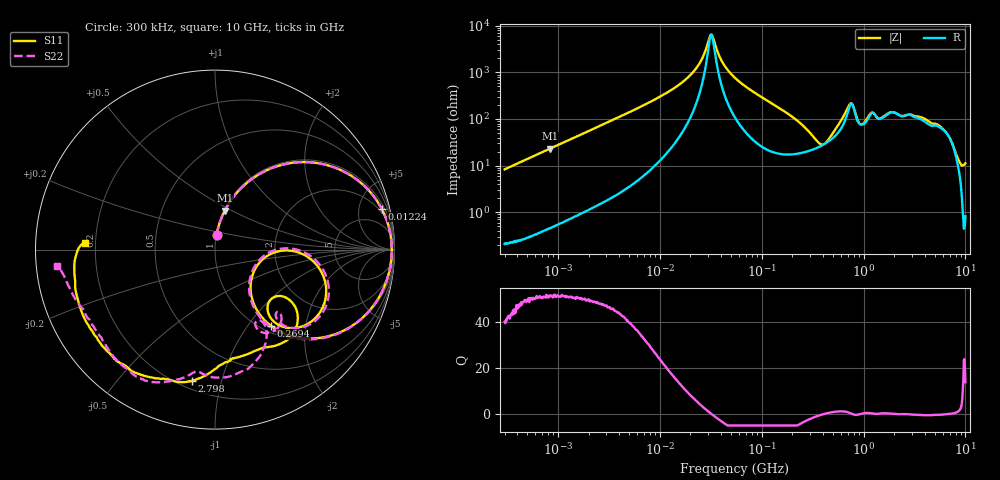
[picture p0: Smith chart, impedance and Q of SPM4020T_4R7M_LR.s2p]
! S-Parameter Data Generated by TDK Corporation
! Copyright(C) 2019 TDK Corporation.
! All Rights Reserved.
! TDK P/N: SPM4020T-4R7M-LR (Inductor)
! Property: L=4.7uH at 100kHz
! Size(LxWxT): 4.4x4.1x2mm
! Model Type: s2p (Touchstone File Format Version 1.0)
! Frequency: DC=Yes Start=0.3MHz Stop=10000MHz 802points Log-sweep
! Model Generated on Sep. 23, 2019
! Port Assignments:
!  1 ---@@@--- 2
! Applicable Conditions:
!  Temperature = 25 degC
!  DC Bias Current = 0 A
!  Small Signal Operation
! Terms and conditions regarding TDK Simulation Models
! (1)This simulation model is being provided solely for informational purposes. Please refer to the specifications of the products in terms of detailed characteristics of such products.
! (2)In no event shall TDK Corporation of any of its subsidiaries be liable for any loss or damage arising, directly or indirectly,
!  From any information contained in this simulation model, including, but not limited to loss or damages arising from any inaccuracies, omissions or errors in connection with such information.
! (3)Any and all copyrights on this simulation model are owned by TDK Corporation.
!  Duplication or redistribution of this simulation model without prior written permission from TDK Corporation is prohibited.
! (4)This simulation model is subject to any modification or change without any prior notice.
! (5)Neither TDK Corporation nor any of its subsidiaries shall make any warranty, express or implied,
!  Including but not limited to the correctness, implied warranties of merchantability and fitness for a particular purpose with respect to this simulation models.
! (6)The use of this simulation model shall be deemed to have consented to the terms and conditions hereof.
# Hz S MA R 50
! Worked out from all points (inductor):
!   801 points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, 300 kHz to 10 GHz, reference 50 ohm
!   read as one part in series: L = 4.4 uH near 318.3 kHz
!   highest Q = 51.2 at 832.9 kHz (marker M1), where L = 4.4 uH
!   self-resonance near 32.06 MHz
!   S11 on the Smith chart (normalised r, x): 300 kHz: 1.00, +0.17; 12.24 MHz: 1.50, +7.98; 269.4 MHz: 1.10, -1.30; 2.798 GHz: 0.25, -0.81; 10 GHz: 0.16, +0.02
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300000  0.08244 83.8  0.9945 -4.8  0.9946 -4.8  0.08211 83.8
832928  0.2231 76.0  0.9704 -12.9  0.9705 -12.9  0.223 75.9
1713600  0.4229 63.8  0.8977 -25.1  0.8978 -25.1  0.4229 63.8
3911703  0.7253 42.1  0.6721 -46.6  0.6722 -46.6  0.7251 42.1
9671944  0.9328 18.5  0.3243 -69.1  0.3243 -69.1  0.9328 18.5
1.224117e7  0.956 13.8  0.2469 -73.1  0.2469 -73.2  0.956 13.8
2.220835e7  0.9824 4.1  0.08621 -76.6  0.08624 -76.7  0.9824 4.0
3.206042e7  0.9848 -1.2  0.01508 -2.2  0.01508 -2.2  0.9848 -1.2
5.477226e7  0.9741 -9.3  0.1273 72.6  0.1273 72.6  0.9741 -9.4
1.608169e8  0.8098 -36.0  0.5049 47.5  0.505 47.5  0.8094 -36.4
2.694285e8  0.5277 -53.7  0.719 20.2  0.719 20.2  0.5257 -54.6
3.126428e8  0.417 -55.3  0.7574 10.4  0.7574 10.4  0.4138 -56.4
4.329008e8  0.2483 -25.3  0.7561 -13.4  0.7561 -13.4  0.2389 -25.6
5.745924e8  0.4302 -1.0  0.6186 -36.5  0.6186 -36.6  0.4213 0.8
7.152593e8  0.6594 -20.0  0.3507 -43.6  0.3507 -43.6  0.662 -17.3
8.299813e8  0.6109 -45.8  0.3926 -12.0  0.3926 -12.0  0.648 -42.1
1.054047e9  0.4489 -35.2  0.4919 -41.1  0.4919 -41.2  0.5061 -44.3
1.228555e9  0.6223 -42.9  0.3648 -42.2  0.3647 -42.2  0.5543 -56.6
1.767019e9  0.6111 -74.7  0.3283 -58.2  0.3283 -58.2  0.6049 -62.8
2.798208e9  0.7424 -100.0  0.2433 -67.1  0.2433 -67.2  0.7134 -101.6
6.172341e9  0.825 -137.1  0.1893 -90.8  0.1894 -90.9  0.8054 -139.3
1e10  0.725 177.3  0.1171 -125.7  0.1172 -125.8  0.8851 -174.2
